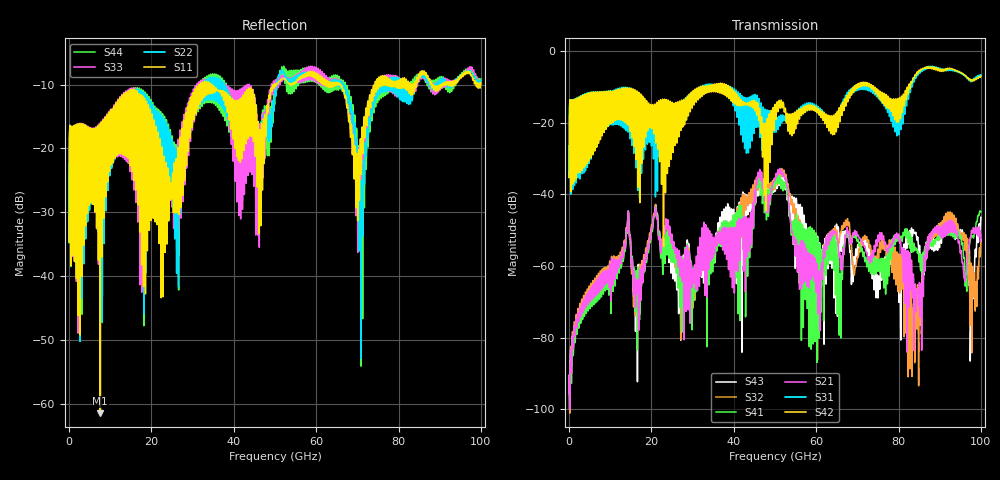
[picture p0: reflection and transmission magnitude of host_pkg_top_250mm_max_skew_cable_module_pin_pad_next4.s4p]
# Hz S RI R 50
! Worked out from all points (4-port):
!   10000 points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, 10 MHz to 100 GHz, reference 50 ohm
!   strongest paths, dB at 10 MHz, 25.01 GHz, 50.01 GHz, 75.01 GHz, 100 GHz:
!     S42: -35.3, -14.4, -15.0, -11.9, -7.0
!     S31: -35.3, -17.3, -18.5, -12.2, -6.7
!     S21: -95.5, -51.5, -35.9, -51.3, -51.2
!     S41: -95.5, -54.0, -36.9, -61.3, -44.8
!     S32: -95.6, -52.8, -38.1, -55.7, -52.6
!     S43: -95.5, -55.4, -38.4, -67.9, -46.4
!   lowest |S11| = -61.5 dB at 7.58 GHz (marker M1), VSWR 1.00, Z = 50 + j0.0833 ohm
!   |S11| at or under -10 dB: start of sweep to 31.5 GHz; 34.77 GHz to 49.48 GHz (14.71 GHz wide, 34.9 % of centre); 65.94 GHz to 74.3 GHz (8.358 GHz wide, 11.9 % of centre)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
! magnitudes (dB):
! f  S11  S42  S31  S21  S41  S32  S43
! 10 MHz  -34.7  -35.3  -35.3  -95.5  -95.5  -95.6  -95.5
! 7.58 GHz  -61.5  -22.4  -24.1  -62.5  -63.7  -61.5  -62.7
! 51.65 GHz  -9.2  -15.0  -20.0  -33.5  -36.0  -32.9  -34.5
! 60.32 GHz  -9.1  -16.9  -15.9  -61.4  -55.0  -86.2  -52.1
! 92.26 GHz  -10.1  -4.9  -5.4  -50.5  -51.3  -47.0  -48.2
! 97.81 GHz  -8.5  -8.1  -8.0  -50.1  -51.5  -72.4  -69.0
! 100 GHz  -9.7  -7.0  -6.7  -51.2  -44.8  -52.6  -46.4
